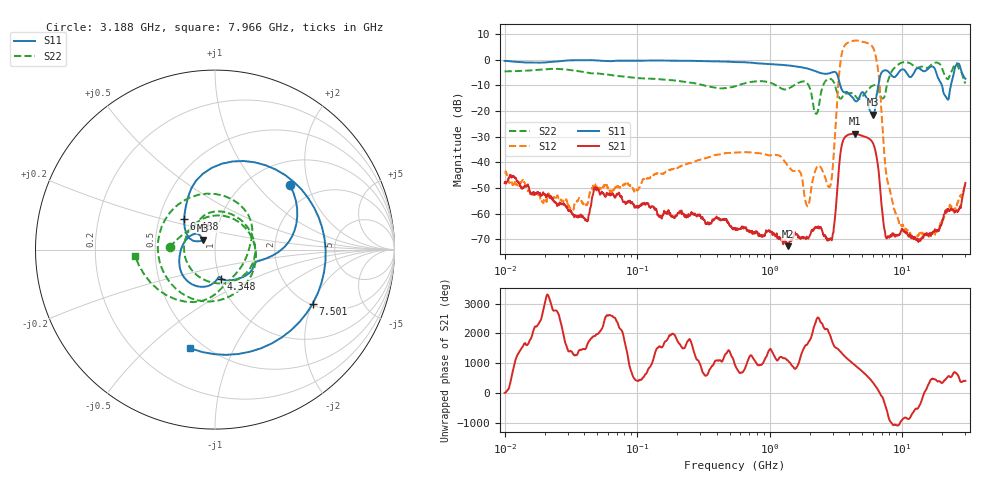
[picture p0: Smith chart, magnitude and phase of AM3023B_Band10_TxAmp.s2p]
# Hz S DB R 50.0
!freq dBS11 angS11 dBS21 angS21 dBS12 angS12 dBS22 angS22
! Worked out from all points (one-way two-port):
!   1601 points, 10 MHz to 30 GHz, reference 50 ohm
!   highest |S21| = -28.84 dB at 4.414 GHz (marker M1); lowest = -72.7 dB at 1.382 GHz (marker M2)
!   lowest |S11| = -21.5 dB at 6.049 GHz (marker M3), VSWR 1.18, Z = 43.7 + j4.74 ohm
!   |S11| at or under -10 dB: 3.408 GHz to 6.623 GHz (3.215 GHz wide, 64.1 % of centre); 19.94 GHz to 23.31 GHz (3.369 GHz wide, 15.6 % of centre)
!   |S22| runs from -21.1 to -0.9 dB; largest |S21 - S12| = 2.4
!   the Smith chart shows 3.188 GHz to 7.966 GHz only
!   S11 on the Smith chart (normalised r, x): 3.188 GHz: 1.48, +1.53; 4.348 GHz: 1.02, -0.34; 6.488 GHz: 0.67, +0.24; 7.501 GHz: 2.05, -2.02; 7.966 GHz: 0.43, -0.69
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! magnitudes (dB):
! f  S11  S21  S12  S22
! 10 MHz  -0.5  -48.1  -44.0  -4.6
! 38.04 MHz  -0.2  -60.5  -55.1  -4.7
! 49.1 MHz  -0.3  -50.6  -49.7  -5.3
! 144.7 MHz  -0.3  -60.4  -44.4  -7.6
! 547.7 MHz  -0.9  -66.1  -36.2  -10.4
! 1.382 GHz  -2.2  -72.7  -41.5  -11.3
! 1.914 GHz  -3.4  -69.2  -56.9  -9.1
! 2.084 GHz  -4.0  -66.3  -48.5  -14.3
! 2.856 GHz  -5.2  -70.0  -49.5  -7.5
! 3.188 GHz  -5.2  -54.9  -20.7  -12.0
! 3.541 GHz  -12.1  -32.3  3.4  -14.4
! 4.348 GHz  -15.6  -28.8  7.4  -13.6
! 4.414 GHz  -16.1  -28.8  7.5  -14.0
! 6.049 GHz  -21.5  -32.8  4.6  -10.1
! 6.488 GHz  -12.4  -39.5  -1.9  -10.2
! 7.501 GHz  -4.1  -69.0  -42.5  -12.7
! 7.926 GHz  -4.8  -69.1  -49.1  -7.3
! 7.966 GHz  -4.9  -69.1  -49.6  -7.0
! 12.43 GHz  -4.6  -69.0  -69.4  -2.7
! 21.67 GHz  -14.9  -59.2  -59.4  -7.3
! 25.95 GHz  -1.6  -59.2  -56.0  -1.6
! 30 GHz  -7.5  -48.1  -48.8  -9.3
